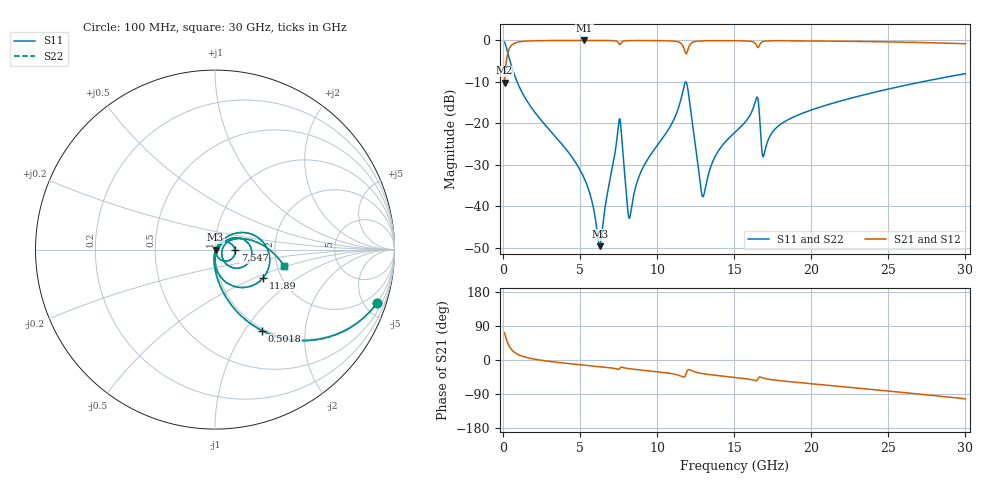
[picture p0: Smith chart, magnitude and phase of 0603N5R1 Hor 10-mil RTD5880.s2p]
# GHz S MA R 50
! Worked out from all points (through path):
!   3201 points, 100 MHz to 30 GHz, reference 50 ohm
!   highest |S21| = -0.03 dB at 5.276 GHz (marker M1); lowest = -10.2 dB at 100 MHz (marker M2)
!   group delay of S21, straight-line fit = 10.4 ps
!   lowest |S11| = -49.6 dB at 6.267 GHz (marker M3), VSWR 1.01, Z = 50.3 - j0.117 ohm
!   |S11| at or under -10 dB: 911.2 MHz to 27.19 GHz (26.28 GHz wide, 187 % of centre)
!   |S22| runs from -49.6 to -0.4 dB; largest |S21 - S12| = 0
!   S11 on the Smith chart (normalised r, x): 100 MHz: 0.97, -6.09; 501.8 MHz: 0.97, -1.21; 7.547 GHz: 1.25, -0.01; 11.89 GHz: 1.62, -0.56; 30 GHz: 2.18, -0.48
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0.1  0.9514 -18.2  0.3078 71.8  0.3078 71.8  0.9514 -18.2
0.5017812  0.5223 -59.8  0.8521 30.1  0.8521 30.1  0.5223 -59.8
1.454844  0.1992 -82.2  0.9787 7.4  0.9787 7.4  0.1992 -82.2
5.089563  0.02538 -97.1  0.9971 -12.8  0.9971 -12.8  0.02538 -97.1
5.276438  0.02148 -96.6  0.9971 -13.5  0.9971 -13.5  0.02148 -96.6
6.266875  0.003297 -20.6  0.9966 -17.5  0.9966 -17.5  0.003297 -20.6
7.546969  0.1119 -2.1  0.8947 -23.4  0.8947 -23.4  0.1119 -2.1
8.201031  0.007155 -5.9  0.993 -23.0  0.993 -23.0  0.007155 -5.9
8.901813  0.02484 52.9  0.9949 -26.2  0.9949 -26.2  0.02484 52.9
10.06978  0.05613 52.8  0.9924 -31.2  0.9924 -31.2  0.05613 52.8
11.52741  0.1902 29.9  0.9254 -42.4  0.9254 -42.4  0.1902 29.9
11.89181  0.3117 -30.1  0.6887 -34.2  0.6887 -34.2  0.3117 -30.1
12.23753  0.1165 -84.6  0.9305 -28.3  0.9305 -28.3  0.1165 -84.6
12.957  0.01302 -25.6  0.987 -35.9  0.987 -35.9  0.01302 -25.6
13.78859  0.04069 39.0  0.9915 -40.3  0.9915 -40.3  0.04069 39.0
15.05  0.07795 39.0  0.9898 -45.8  0.9898 -45.8  0.07795 39.0
16.45156  0.2034 -0.4  0.8669 -54.6  0.8669 -54.6  0.2034 -0.4
16.92809  0.04165 4.7  0.9741 -48.2  0.9741 -48.2  0.04165 4.7
17.79706  0.09058 31.5  0.9882 -53.8  0.9882 -53.8  0.09058 31.5
20.03956  0.1453 24.9  0.9832 -62.8  0.9832 -62.8  0.1453 24.9
25.01978  0.2593 6.5  0.9588 -82.0  0.9588 -82.0  0.2593 6.5
30  0.3967 -13.5  0.9098 -102.4  0.9098 -102.4  0.3967 -13.5
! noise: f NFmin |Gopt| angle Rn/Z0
0.1  0.0003794  0.9372  0.6569  0.001348
3.417  0.003834  0.8009  9.673  0.003965
6.743  0.008023  0.812  18.82  0.008668
10.06  0.01129  0.8031  27.88  0.01122
13.39  0.01608  0.8166  36.92  0.01652
16.7  0.05507  0.9298  45.75  0.1479
20.03  0.01594  0.7408  54  0.00984
23.35  0.01784  0.7347  62.17  0.009932
26.67  0.02018  0.7358  70.14  0.01034
30  0.0228  0.7401  77.89  0.01079
